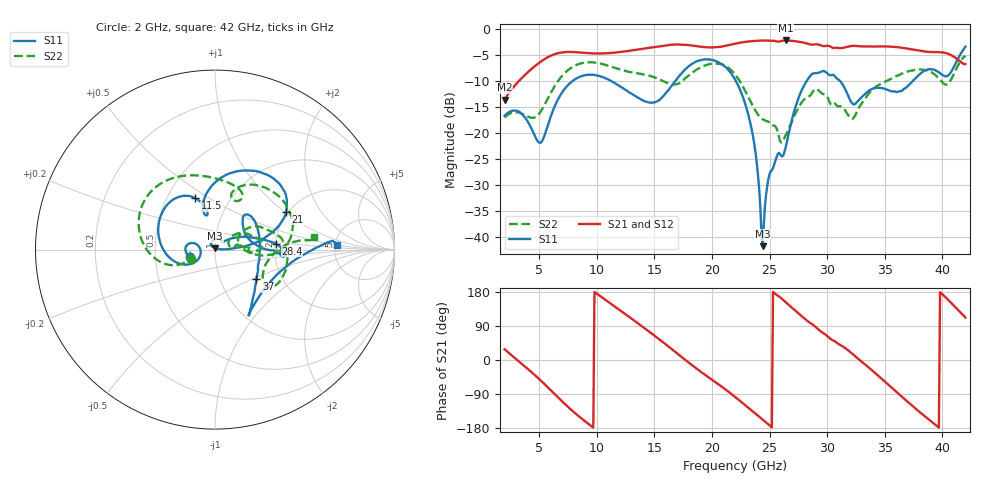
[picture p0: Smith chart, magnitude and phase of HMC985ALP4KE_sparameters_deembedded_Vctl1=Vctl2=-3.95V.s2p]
!s2p File: Measurements: S11, S21, S12, S22
# GHz S dB R 50.0
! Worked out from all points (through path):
!   401 points, 2 GHz to 42 GHz, reference 50 ohm
!   highest |S21| = -2.16 dB at 26.4 GHz (marker M1); lowest = -13.6 dB at 2 GHz (marker M2)
!   lowest |S11| = -41.8 dB at 24.4 GHz (marker M3), VSWR 1.02, Z = 50.1 + j0.811 ohm
!   |S11| at or under -10 dB: start of sweep to 7.883 GHz; 22.09 GHz to 28.22 GHz (6.129 GHz wide, 24.4 % of centre); 31.13 GHz to 37.41 GHz (6.285 GHz wide, 18.3 % of centre)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
!   |S22| runs from -21.8 to -5.1 dB; largest |S21 - S12| = 0.00063
!   S11 on the Smith chart (normalised r, x): 2 GHz: 0.75, -0.06; 11.5 GHz: 0.69, +0.44; 21 GHz: 1.95, +1.03; 28.4 GHz: 2.01, +0.15; 37 GHz: 1.48, -0.53; 42 GHz: 5.22, +0.50
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2  -16.65 -163.9  -13.55 28.3  -13.55 28.3  -17.00 -158.2
3.4  -16.12 170.0  -9.60 -7.8  -9.60 -7.8  -16.17 -176.1
5.1  -21.86 -171.5  -6.30 -53.1  -6.30 -53.1  -15.95 -160.4
6.3  -15.09 -151.7  -4.83 -88.5  -4.83 -88.6  -11.12 -162.6
8.7  -9.02 149.7  -4.50 -155.0  -4.50 -155.0  -6.52 150.7
11.5  -10.28 110.8  -4.51 142.4  -4.52 142.4  -7.38 104.5
13.6  -13.22 101.7  -3.89 96.2  -3.89 96.2  -8.51 75.3
15.4  -13.68 106.6  -3.30 55.2  -3.30 55.2  -9.63 62.4
17.9  -7.27 79.0  -3.04 -5.0  -3.04 -5.0  -9.05 71.6
21  -6.96 28.1  -3.26 -73.7  -3.26 -73.7  -6.87 16.9
22  -9.63 16.5  -2.78 -97.2  -2.78 -97.2  -8.67 -0.2
23.5  -19.84 3.8  -2.29 -134.6  -2.28 -134.6  -14.58 -4.3
24.4  -41.78 83.7  -2.18 -157.3  -2.18 -157.3  -17.32 8.9
25  -27.88 124.7  -2.20 -172.6  -2.20 -172.6  -17.94 12.4
26.4  -22.72 41.2  -2.16 152.5  -2.15 152.6  -20.44 34.0
28.4  -9.38 5.6  -2.85 100.4  -2.84 100.4  -12.95 17.2
28.7  -8.60 0.7  -2.98 94.3  -2.98 94.3  -12.22 15.5
32.4  -14.41 31.0  -3.20 10.6  -3.20 10.6  -16.72 27.0
35.4  -11.78 16.8  -3.33 -67.5  -3.32 -67.4  -9.72 18.3
37  -10.94 -35.7  -3.74 -110.6  -3.74 -110.6  -8.13 3.5
39.8  -8.46 -55.1  -4.42 179.0  -4.42 179.0  -9.75 -33.5
42  -3.34 2.2  -6.69 111.6  -6.69 111.6  -5.07 7.2
